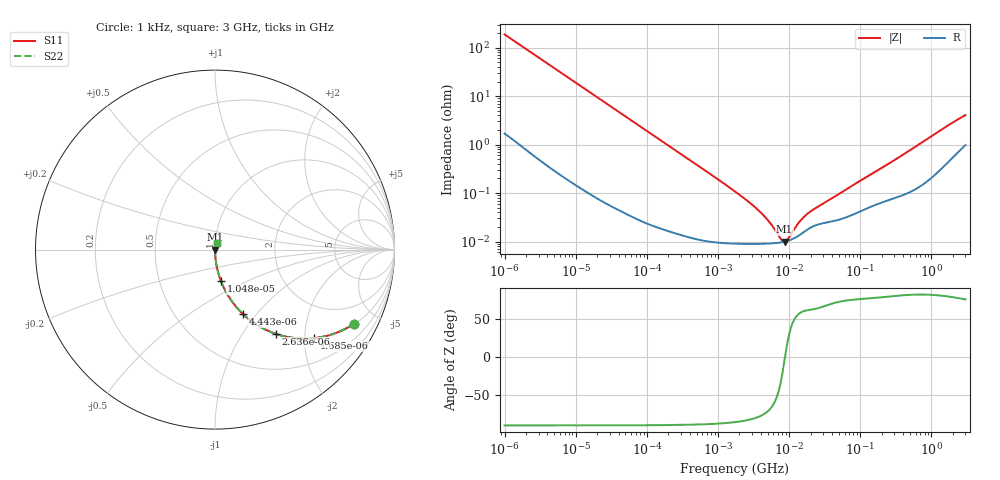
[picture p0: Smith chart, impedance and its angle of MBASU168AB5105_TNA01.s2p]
! MBASU168AB5105_TNA01  S-PARAMETER MODEL  ( Standard Model )
! Model Generated by TAIYO YUDEN Corporation (http://www.ty-top.com)
! Version 1.0
! TAIYO YUDEN Control No. 220601
! Copyright(c) 2012 TAIYO YUDEN CO.,LTD. All Rights Reserved.
! Product Description (link to TY-COMPAS)
! https://ds.yuden.co.jp/TYCOMPAS/or/detail?pn=MBASU168AB5105KTNA01&u=M
! Products Name : Multilayer Ceramic Capacitors
! Characteristics :
!  Capacitance : 1 [uF] , Rated Voltage : 50 [V] , TCC : X5R
!  Case Size : 1.6 x 0.8 / 0.063 x 0.031 [mm/inch] , Thickness : 0.8 / 0.031 [mm/inch]
!  (Conditions: Temperature = 25 [degC] , DC Bias Voltage = 0 [V])
! External Node Assignments :
!  1  o---| |---o  2
! GND o---------o GND
! Frequency Range : 1kHz  -  3GHz  [ 401 STEP ]
# MHZ S RI R 50
! Freq[MHz].  S11 Real  S11 Imag  S21 Real  S21 Imag  S12 Real  S12 Imag  S22 Real  S22 Imag
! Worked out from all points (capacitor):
!   401 points, 1 kHz to 3 GHz, reference 50 ohm
!   read as one part in series: C = 848 nF near 1.077 kHz
!   lowest |Z| = 9.94 mohm at 8.607 MHz (marker M1)
!   series resonance near 8.729 MHz, so ESL is about 390 pH
!   S11 on the Smith chart (normalised r, x): 1 kHz: 1.03, -3.75; 1.685 kHz: 1.02, -2.23; 2.636 kHz: 1.01, -1.43; 4.443 kHz: 1.01, -0.85; 10.47 kHz: 1.00, -0.36; 3 GHz: 1.02, +0.08
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0.001  0.7762 -0.4123  0.2238 0.4123  0.2238 0.4123  0.7762 -0.4123
0.001685  0.5539 -0.4929  0.4461 0.4929  0.4461 0.4929  0.5539 -0.4929
0.002636  0.3393 -0.4695  0.6607 0.4695  0.6607 0.4695  0.3393 -0.4695
0.004443  0.1549 -0.358  0.8451 0.358  0.8451 0.358  0.1549 -0.358
0.006451  0.0809 -0.2689  0.9191 0.2689  0.9191 0.2689  0.0809 -0.2689
0.010475  0.033 -0.1748  0.967 0.1748  0.967 0.1748  0.033 -0.1748
0.01216  0.0249 -0.1519  0.9751 0.1519  0.9751 0.1519  0.0249 -0.1519
0.033275  0.00377 -0.057  0.9962 0.057  0.9962 0.057  0.00377 -0.057
0.147855  0.000358 -0.013  0.9996 0.013  0.9996 0.013  0.000358 -0.013
1.732051  9.15e-05 -0.00108  0.9999 0.00108  0.9999 0.00108  9.15e-05 -0.00108
2.812335  8.96e-05 -0.00062  0.9999 0.00062  0.9999 0.00062  8.96e-05 -0.00062
4.083148  8.98e-05 -0.000373  0.9999 0.000373  0.9999 0.000373  8.98e-05 -0.000373
5.502215  9.13e-05 -0.000214  0.9999 0.000214  0.9999 0.000214  9.13e-05 -0.000214
7.696136  9.61e-05 -5.69e-05  0.9999 5.69e-05  0.9999 5.69e-05  9.61e-05 -5.69e-05
8.606987  9.92e-05 -6.31e-06  0.9999 6.31e-06  0.9999 6.31e-06  9.92e-05 -6.31e-06
9.625639  0.000104 4.44e-05  0.9999 -4.44e-05  0.9999 -4.44e-05  0.000104 4.44e-05
12.49624  0.000123 0.000164  0.9999 -0.000164  0.9999 -0.000164  0.000123 0.000164
15.05716  0.000146 0.00025  0.9999 -0.00025  0.9999 -0.00025  0.000146 0.00025
21.06097  0.000201 0.000393  0.9998 -0.000393  0.9998 -0.000393  0.000201 0.000393
256.0921  0.000738 0.00405  0.9993 -0.00405  0.9993 -0.00405  0.000738 0.00405
1652.1  0.00465 0.0235  0.9953 -0.0235  0.9953 -0.0235  0.00465 0.0235
3000  0.0112 0.0387  0.9888 -0.0387  0.9888 -0.0387  0.0112 0.0387
